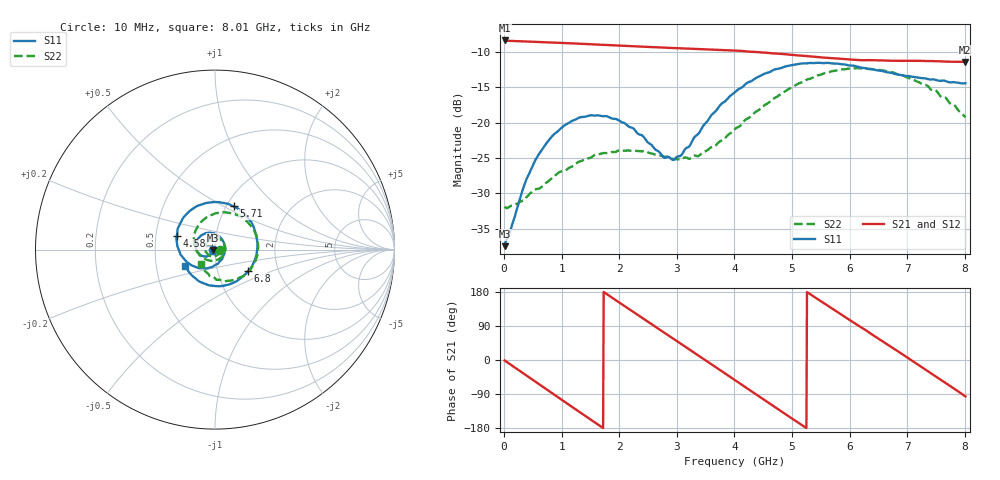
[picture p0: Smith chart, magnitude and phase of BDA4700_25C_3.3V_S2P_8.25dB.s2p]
!Agilent Technologies,E5071B,MY42404982,A.09.10
!Date: Mon Oct 20 18:06:27 2025
!Data & Calibration Information:
!Freq	S11:SOLT2(ON)	S21:SOLT2(ON)	S12:SOLT2(ON)	S22:SOLT2(ON)
# Hz S RI R 50
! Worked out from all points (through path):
!   801 points, 10 MHz to 8.01 GHz, reference 50 ohm
!   highest |S21| = -8.37 dB at 20 MHz (marker M1); lowest = -11.4 dB at 8 GHz (marker M2)
!   group delay of S21, straight-line fit = 282 ps
!   lowest |S11| = -37.5 dB at 10 MHz (marker M3), VSWR 1.03, Z = 48.7 - j0.158 ohm
!   |S11| at or under -10 dB: start of sweep to end of sweep
!   |S22| runs from -32.1 to -12.3 dB; largest |S21 - S12| = 0.0043
!   S11 on the Smith chart (normalised r, x): 10 MHz: 0.97, -0.00; 4.58 GHz: 0.64, +0.10; 5.71 GHz: 1.08, +0.56; 6.8 GHz: 1.40, -0.35; 8.01 GHz: 0.70, -0.13
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1e7  -0.0133 -0.00162  0.3814 -0.00822  0.3813 -0.0087  0.0254 -0.00138
2e7  -0.0138 -0.00253  0.3813 -0.0152  0.3812 -0.0162  0.0251 -0.00138
5.8e8  -0.0435 -0.0378  0.1792 -0.3264  0.1791 -0.3266  0.0109 -0.0322
9.5e8  -0.0838 -0.0275  -0.0624 -0.362  -0.0622 -0.362  -0.0235 -0.0376
1.35e9  -0.1078 0.0197  -0.2818 -0.226  -0.2819 -0.2262  -0.0534 -0.00507
1.93e9  -0.0567 0.09  -0.3284 0.1266  -0.3285 0.1268  -0.0237 0.0573
2.32e9  0.00682 0.0834  -0.1679 0.3022  -0.1677 0.3022  0.0268 0.0571
2.68e9  0.0496 0.0383  0.0454 0.338  0.0449 0.3377  0.056 0.0177
2.95e9  0.0532 -0.0129  0.1939 0.2759  0.1935 0.2753  0.052 -0.0183
3.37e9  0.00754 -0.0828  0.3243 0.0702  0.3247 0.0703  0.0101 -0.057
3.68e9  -0.0623 -0.104  0.309 -0.1086  0.309 -0.1096  -0.0363 -0.0589
4.01e9  -0.1447 -0.0779  0.1937 -0.259  0.1941 -0.2584  -0.0834 -0.0335
4.58e9  -0.2129 0.075  -0.1148 -0.2897  -0.1143 -0.2901  -0.1156 0.0739
4.98e9  -0.1562 0.2006  -0.2672 -0.1404  -0.2676 -0.1417  -0.069 0.1621
5.35e9  -0.0342 0.2619  -0.2894 0.0496  -0.2897 0.0479  0.0282 0.2049
5.71e9  0.1032 0.241  -0.1999 0.2041  -0.1996 0.2041  0.1401 0.1845
6.18e9  0.222 0.1061  0.00898 0.2767  0.0117 0.2774  0.2338 0.0624
6.68e9  0.2112 -0.0816  0.2146 0.1711  0.2152 0.1709  0.2089 -0.0914
6.8e9  0.1855 -0.1193  0.2447 0.1234  0.2456 0.1216  0.1877 -0.1199
7.33e9  0.0174 -0.2043  0.244 -0.122  0.2441 -0.1227  0.0515 -0.1768
8e9  -0.1656 -0.0922  -0.023 -0.2679  -0.0225 -0.2683  -0.075 -0.081
8.01e9  -0.1674 -0.0898  -0.028 -0.2675  -0.0268 -0.2676  -0.0757 -0.0786
